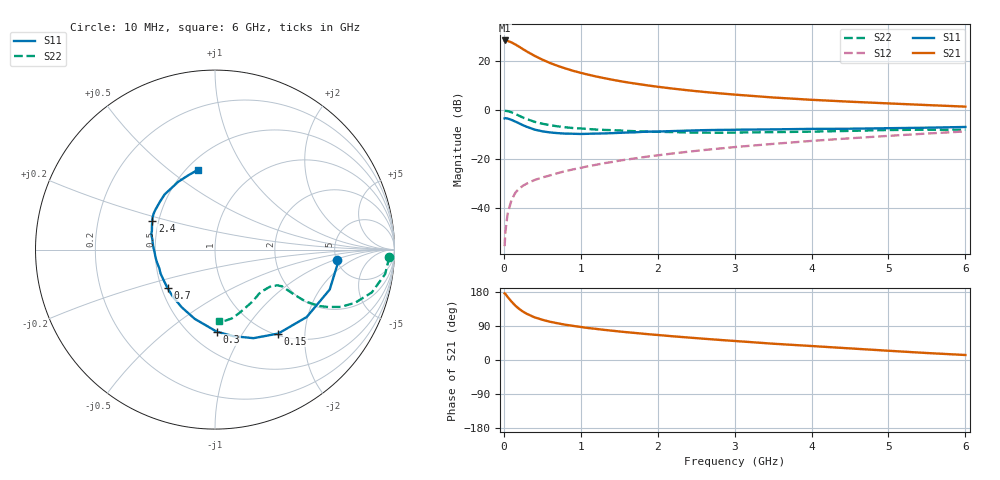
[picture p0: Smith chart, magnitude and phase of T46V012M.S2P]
! Infineon Technologies  Discrete & RF Semiconductors
! BFR182T
! Si NPN RF Bipolar Junction Transistor in SC75
! VCE = 6 V  IC = 12 mA
! Common Emitter S-Parameters:  October  1999
# GHz  S  MA  R  50
!  f  S11  S21  S12  S22
! GHz  MAG  ANG  MAG  ANG  MAG  ANG  MAG  ANG
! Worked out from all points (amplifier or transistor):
!   36 points, 10 MHz to 6 GHz, reference 50 ohm
!   highest |S21| = 28.4 dB at 10 MHz (marker M1)
!   |S21| within 3 dB of that: start of sweep to 221.9 MHz
!   unconditionally stable (mu >= 1): 968.2 MHz to 3.845 GHz
!   at 250 MHz: K = 0.48, MSG = 27.8 dB, |S12| = -30.8 dB
!   at 1.4 GHz: K = 1.07, MAG = 15.2 dB, |S12| = -21.1 dB
!   at 6 GHz: K = 0.86, MSG = 5.1 dB, |S12| = -8.6 dB
!   S11 on the Smith chart (normalised r, x): 10 MHz: 5.01, -1.06; 150 MHz: 1.03, -1.47; 300 MHz: 0.67, -0.77; 700 MHz: 0.54, -0.26; 2.4 GHz: 0.46, +0.17; 6 GHz: 0.57, +0.64
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0.01  0.6798 -4.8  26.31 175.8  0.0017 78.5  0.9691 -2.4
0.02  0.6888 -6.2  26.28 174.4  0.0033 95.9  0.9696 -3.3
0.05  0.6767 -19.2  25.71 166.2  0.0079 84.1  0.9575 -8.2
0.1  0.6342 -36.3  24 154.2  0.0149 74.5  0.9054 -15.3
0.15  0.5857 -53.0  21.8 143.3  0.0209 69.1  0.8347 -20.8
0.2  0.5381 -66.5  19.59 134.7  0.0254 65.5  0.7698 -24.5
0.25  0.493 -78.0  17.46 127.6  0.029 62.7  0.7064 -26.9
0.3  0.4577 -88.7  15.64 121.7  0.0321 61.4  0.6583 -28.5
0.4  0.4021 -106.3  12.79 112.6  0.0379 60.3  0.5794 -29.8
0.5  0.371 -120.0  10.71 106.2  0.0426 60.5  0.5305 -29.7
0.6  0.3525 -131.5  9.143 100.9  0.0469 61.7  0.4949 -29.5
0.7  0.3408 -140.8  7.995 96.8  0.0522 62.2  0.468 -29.2
0.9  0.3314 -156.2  6.344 90.0  0.0622 64.3  0.4329 -29.0
1.1  0.331 -167.6  5.273 84.3  0.0725 65.3  0.4131 -29.3
1.3  0.3364 -176.7  4.51 79.6  0.083 66.3  0.3966 -30.2
1.6  0.3505 172.8  3.7 73.3  0.0988 66.8  0.3793 -32.1
2.2  0.3757 159.2  2.746 62.5  0.1316 66.8  0.358 -38.2
2.4  0.3839 155.7  2.533 59.3  0.1427 66.8  0.3515 -40.6
3.5  0.4068 138.8  1.814 43.0  0.2058 63.2  0.3572 -54.8
4.5  0.4192 126.0  1.489 30.6  0.2676 58.7  0.3789 -69.3
5.5  0.4399 109.8  1.272 18.4  0.3342 53.3  0.4001 -81.7
6  0.4551 101.9  1.182 13.2  0.3695 49.7  0.4005 -86.6
